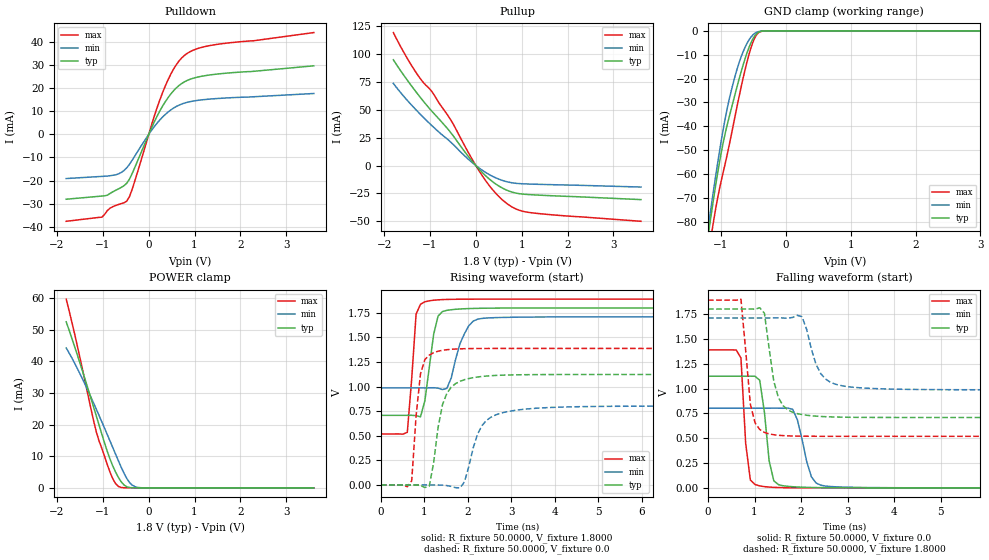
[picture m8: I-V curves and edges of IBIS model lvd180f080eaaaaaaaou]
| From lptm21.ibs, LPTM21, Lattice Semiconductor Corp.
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|   Model lvd180f080eaaaaaaaou
[Model]   lvd180f080eaaaaaaaou
Model_type   Output
Polarity   Non-Inverting
Enable   Active-Low
Vmeas =   0.9000V
Cref =   0.0F
Rref =   1.0000M
Vref =   0.0V
C_comp   4.2000pF   3.8000pF   7.5000pF
[Temperature Range]   25.0000   0.1050k   -40.0000
[Voltage Range]   1.8000V   1.7100V   1.8900V
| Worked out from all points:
|   slope of the pulldown table from 0 to 0.27 V, typ, clamps not added: 24.3 ohm
|   slope of the pullup table from 0 to 0.27 V, typ, clamps not added: 24.1 ohm
|   GND clamp passes 1 mA (typ) near -0.44 V on its own axis
|   POWER clamp passes 1 mA (typ) near -0.54 V on its own axis
|   rising waveform, R_fixture 50.0000, V_fixture 1.8000: 20-80 % time 208ps typ, 314ps min, 136ps max; typ from 0.708 V to 1.8 V
|   rising waveform, R_fixture 50.0000, V_fixture 0.0: 20-80 % time 276ps typ, 394ps min, 161ps max; typ from 0 V to 1.12 V
|   falling waveform, R_fixture 50.0000, V_fixture 0.0: 20-80 % time 168ps typ, 247ps min, 125ps max; typ from 1.12 V to 0 V
|   falling waveform, R_fixture 50.0000, V_fixture 1.8000: 20-80 % time 240ps typ, 322ps min, 173ps max; typ from 1.8 V to 0.708 V
[Pulldown]
|Voltage   I(typ)   I(min)   I(max)
-1.8V     -28.04mA   -19.11mA   -37.59mA
-1.02V    -26.67mA   -18.17mA   -35.8mA
-840mV    -25.49mA   -17.88mA   -31.86mA
-660mV    -23.57mA   -17.1mA    -30.33mA
-480mV    -21.13mA   -14.49mA   -28.87mA
-360mV    -16.89mA   -11.13mA   -23.66mA
120mV     5.351mA    3.322mA    7.82mA
300mV     12.14mA    7.44mA     17.93mA
540mV     18.82mA    11.34mA    28.16mA
780mV     22.73mA    13.53mA    34.14mA
1.38V     25.81mA    15.33mA    38.55mA
3.6V      29.63mA    17.66mA    44.01mA
[Pullup]
|Voltage   I(typ)   I(min)   I(max)
-1.8V     94.9mA     73.7mA     119.3mA
-1.56V    80.29mA    61.51mA    100.7mA
-1.32V    66.89mA    50.65mA    84.45mA
-1.14V    57.49mA    43.08mA    74.2mA
-960mV    48.77mA    35.87mA    66.46mA
-540mV    29.18mA    20.75mA    40.47mA
-120mV    5.911mA    4.081mA    8.509mA
300mV     -12.3mA    -8.255mA   -18.3mA
660mV     -21.81mA   -14.3mA    -33.54mA
900mV     -24.89mA   -16.01mA   -39.35mA
1.2V      -26.11mA   -16.61mA   -42.25mA
3.6V      -30.51mA   -19.25mA   -49.97mA
[GND_clamp]
|Voltage   I(typ)   I(min)   I(max)
-1.8V     -240.2mA   -229.4mA   -254.3mA
-1.2V     -86.16mA   -82.91mA   -94.88mA
-1.17V    -80.45mA   -77.09mA   -89.3mA
-1.11V    -69.45mA   -65.77mA   -78.87mA
-1.02V    -54.48mA   -49.86mA   -65.69mA
-930mV    -42.25mA   -35.9mA    -54.92mA
-780mV    -26.14mA   -18.58mA   -35.25mA
-690mV    -17.13mA   -10.87mA   -23.53mA
-570mV    -7.024mA   -3.834mA   -9.978mA
-450mV    -1.176mA   -584.6uA   -1.582mA
-300mV    -18.65uA   -15.9uA    -16.44uA
3.6V      0A         0A         0A
[POWER_clamp]
|Voltage   I(typ)   I(min)   I(max)
-1.8V     52.51mA    44.24mA    59.69mA
-1.68V    47.44mA    41.17mA    52.62mA
-1.5V     39.45mA    36.1mA     41.14mA
-1.26V    28.3mA     28.66mA    24.99mA
-1.14V    22.57mA    24.76mA    17.52mA
-840mV    8.928mA    14.66mA    4.779mA
-720mV    4.91mA     10.55mA    1.28mA
-660mV    3.265mA    8.507mA    435.9uA
-540mV    921.6uA    4.64mA     35.01uA
-420mV    115.2uA    1.718mA    2.184uA
-240mV    3.289uA    139.9uA    57.44nA
3.6V      -31nA      -27.04nA   -40.53nA
[Ramp]
| variable   typ   min   max
dV/dt_r  0.6610/0.2727n   0.4811/0.3898n   0.8331/0.1596n
dV/dt_f  0.6551/0.2377n   0.4337/0.3185n   0.8227/0.1714n
R_load = 50.0000
[Rising Waveform]
R_fixture=   50.0000
V_fixture=   1.8000
V_fixture_min=   1.7100
V_fixture_max=   1.8900
|time   V(typ)   V(min)   V(max)
0s        708.2mV    987.1mV    518.8mV
606.1ps   708.2mV    987.1mV    535.6mV
808.1ps   705.1mV    987.1mV    1.738V
1.01ns    857.5mV    987.1mV    1.863V
1.212ns   1.533V     988.7mV    1.879V
1.313ns   1.717V     984.6mV    1.883V
1.515ns   1.776V     982.4mV    1.887V
1.818ns   1.79V      1.438V     1.889V
2.222ns   1.796V     1.686V     1.89V
10ns      1.8V       1.71V      1.89V
[Rising Waveform]
R_fixture=   50.0000
V_fixture=   0.0
V_fixture_min=   0.0
V_fixture_max=   0.0
|time   V(typ)   V(min)   V(max)
0s        416.8nV    613.5nV    315.6nV
707.1ps   -43.83uV   739.1nV    42.13mV
909.1ps   -4.797mV   13.25uV    1.131V
1.111ns   -12.22mV   23.29uV    1.321V
1.313ns   582.7mV    -542uV     1.36V
1.717ns   1.031V     -27.73mV   1.383V
1.919ns   1.071V     30.53mV    1.386V
2.323ns   1.103V     603.9mV    1.388V
2.929ns   1.118V     747.5mV    1.388V
10ns      1.124V     801.8mV    1.389V
[Falling Waveform]
R_fixture=   50.0000
V_fixture=   0.0
V_fixture_min=   0.0
V_fixture_max=   0.0
|time   V(typ)   V(min)   V(max)
0s        1.124V     801.8mV    1.389V
707.1ps   1.124V     801.8mV    1.307V
808.1ps   1.124V     801.8mV    450.3mV
1.01ns    1.123V     801.8mV    33.5mV
1.111ns   1.083V     801.8mV    19.63mV
1.313ns   272.3mV    801.9mV    7.872mV
1.515ns   31.84mV    802.1mV    3.154mV
1.818ns   11.39mV    791mV      801.3uV
2.424ns   2.244mV    27.1mV     89.53uV
10ns      8.255uV    -8.342uV   -6.339uV
[Falling Waveform]
R_fixture=   50.0000
V_fixture=   1.8000
V_fixture_min=   1.7100
V_fixture_max=   1.8900
|time   V(typ)   V(min)   V(max)
0s        1.8V       1.71V      1.89V
707.1ps   1.8V       1.71V      1.9V
909.1ps   1.801V     1.71V      842.5mV
1.212ns   1.758V     1.71V      558mV
1.313ns   1.403V     1.71V      543.3mV
1.515ns   905.4mV    1.711V     529mV
2.02ns    737.8mV    1.722V     520.2mV
2.424ns   718.8mV    1.149V     519.1mV
2.828ns   712.1mV    1.032V     518.9mV
10ns      708.2mV    987.1mV    518.8mV
